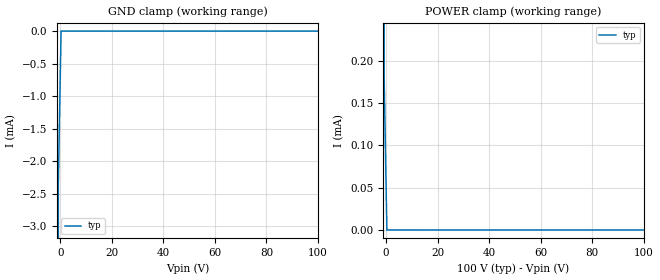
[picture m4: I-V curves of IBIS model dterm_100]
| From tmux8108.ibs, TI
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| dterm_100
[Model]   dterm_100
Model_type   Terminator
|   typ   min   max
C_comp   1.008417e-11   NA   NA
[Voltage Range]   100   NA   NA
[Temperature Range]   27   NA   NA
[Power Clamp Reference]   100   NA   NA
[GND Clamp Reference]   0   NA   NA
[GND Clamp]
|   Voltage   I(typ)   I(min)   I(max)
-5V       -4.511A    NA         NA
-1.818V   -457.9mA   NA         NA
-757.6mV  -2.353mA   NA         NA
303mV     -674.4pA   NA         NA
100V      5.811nA    NA         NA
[POWER Clamp]
|   Voltage   I(typ)   I(min)   I(max)
-5V       1.488A     NA         NA
-1.818V   290.8mA    NA         NA
-758mV    181uA      NA         NA
303mV     5.798nA    NA         NA
100V      -717.1pA   NA         NA
